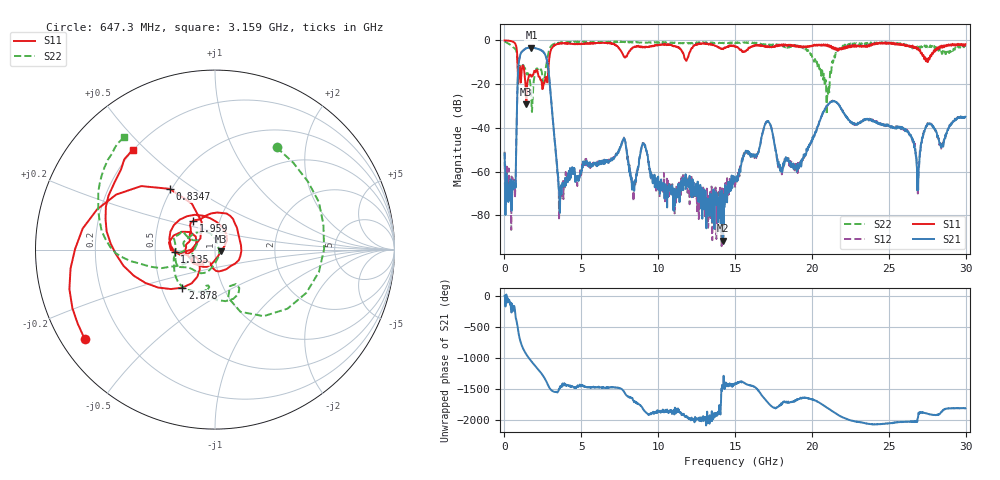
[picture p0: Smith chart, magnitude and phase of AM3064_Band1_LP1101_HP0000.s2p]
# Hz S DB R 50.0
!freq dBS11 angS11 dBS21 angS21 dBS12 angS12 dBS22 angS22
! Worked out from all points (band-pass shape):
!   1600 points, 10 MHz to 29.98 GHz, reference 50 ohm
!   highest |S21| = -3.25 dB at 1.753 GHz (marker M1); lowest = -91.5 dB at 14.2 GHz (marker M2)
!   |S21| within 3 dB of the highest: 1.045 GHz to 2.627 GHz (1.581 GHz wide, 86.1 % of centre)
!   lowest |S11| = -29.2 dB at 1.416 GHz (marker M3), VSWR 1.07, Z = 53.4 - j1.07 ohm
!   |S11| at or under -10 dB: 848.8 MHz to 2.892 GHz (2.043 GHz wide, 109 % of centre)
!   |S22| runs from -33.9 to -0.4 dB; largest |S21 - S12| = 0.0093
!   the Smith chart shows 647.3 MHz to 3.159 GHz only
!   S11 on the Smith chart (normalised r, x): 647.3 MHz: 0.07, -0.31; 834.7 MHz: 0.49, +0.40; 1.135 GHz: 0.63, -0.02; 1.959 GHz: 0.75, +0.25; 2.878 GHz: 0.64, -0.29; 3.159 GHz: 0.20, +0.46
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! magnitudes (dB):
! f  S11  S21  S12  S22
! 10 MHz  0.0  -51.7  -50.9  -0.4
! 647.3 MHz  -1.1  -67.3  -65.1  -3.5
! 834.7 MHz  -7.5  -24.8  -24.7  -8.5
! 1.135 GHz  -13.0  -5.2  -5.1  -12.4
! 1.416 GHz  -29.2  -3.6  -3.5  -15.4
! 1.753 GHz  -16.5  -3.3  -3.2  -27.0
! 1.959 GHz  -13.9  -3.5  -3.4  -16.3
! 2.878 GHz  -11.1  -14.6  -14.6  -5.2
! 3.159 GHz  -2.8  -37.0  -37.1  -1.9
! 3.628 GHz  -1.4  -70.2  -72.5  -1.2
! 5.015 GHz  -1.6  -59.8  -59.0  -0.7
! 7.751 GHz  -7.2  -44.9  -45.2  -0.7
! 10 GHz  -2.1  -62.3  -64.6  -0.9
! 14.2 GHz  -3.9  -91.5  -70.6  -1.1
! 15 GHz  -2.9  -64.1  -67.3  -1.4
! 17.09 GHz  -2.6  -37.0  -37.2  -2.0
! 17.95 GHz  -2.4  -58.3  -59.3  -2.0
! 19.99 GHz  -2.7  -45.8  -45.7  -7.0
! 20.98 GHz  -2.1  -29.9  -29.9  -26.3
! 25 GHz  -1.0  -39.3  -38.9  -1.2
! 26.89 GHz  -3.8  -62.7  -70.0  -3.3
! 29.98 GHz  -1.8  -34.9  -35.0  -2.8
